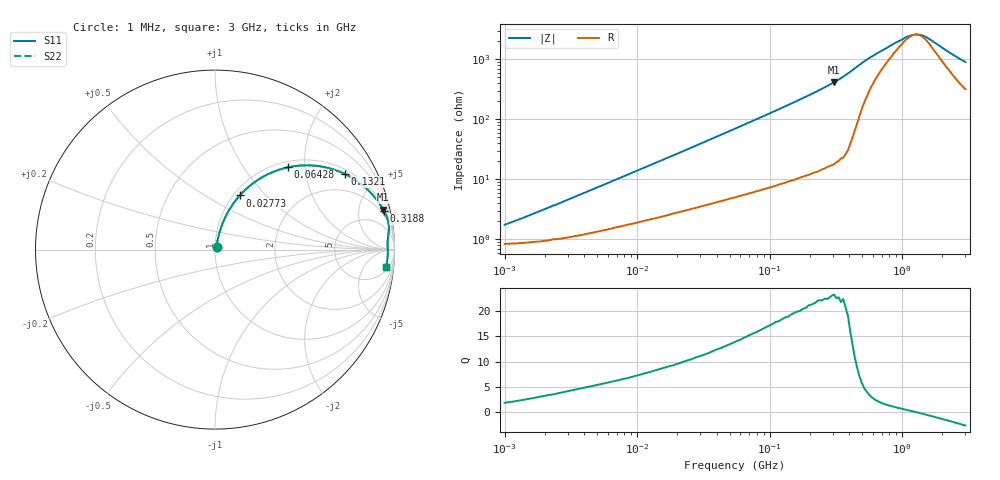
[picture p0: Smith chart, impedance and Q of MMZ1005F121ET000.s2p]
! S-parameter Generated by TDK Corporation
! Copyright(C) 2016 TDK Corporation.
! All Rights Reserved.
! TDK P/N: MMZ1005F121ET000 (Chip Beads)
! Property: |Z|=120¶ at 100MHz
! Size(LxWxT): 1x0.5x0.5mm, 0.039x0.02x0.02inches
! Model Type: s2p (Touchstone File Format Version 1.0)
! Frequency: DC=Yes Start=1MHz Stop=3000MHz 202points Log-sweep
! Note: This model was converted from impedance.
! Model Generated on May. 16, 2016
! Hash(MD5):
! Port Assignments:
!  1 ---@@@--- 2
! Applicable Conditions:
!  Temperature = 25 degC
!  DC Bias Current = 0 A
!  Small Signal Operation
! Terms and conditions regarding TDK Simulation Models
! (1)This simulation model is being provided solely for informational purposes. Please refer to the specifications of the products in terms of detailed characteristics of such products.
! (2)In no event shall TDK Corporation of any of its subsidiaries be liable for any loss or damage arising, directly or indirectly,
!  From any information contained in this simulation model, including, but not limited to loss or damages arising from any inaccuracies, omissions or errors in connection with such information.
! (3)Any and all copyrights on this simulation model are owned by TDK Corporation.
!  Duplication or redistribution of this simulation model without prior written permission from TDK Corporation is prohibited.
! (4)This simulation model is subject to any modification or change without any prior notice.
! (5)Neither TDK Corporation nor any of its subsidiaries shall make any warranty, express or implied,
!  Including but not limited to the correctness, implied warranties of merchantability and fitness for a particular purpose with respect to this simulation models.
! (6)The use of this simulation model shall be deemed to have consented to the terms and conditions hereof.
# MHz S MA R 50
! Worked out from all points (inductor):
!   201 points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, 1 MHz to 3 GHz, reference 50 ohm
!   read as one part in series: L = 240 nH near 1.823 MHz
!   highest Q = 22.7 at 306.3 MHz (marker M1), where L = 216 nH
!   self-resonance near 1.266 GHz
!   S11 on the Smith chart (normalised r, x): 1 MHz: 1.02, +0.03; 27.73 MHz: 1.07, +0.72; 64.28 MHz: 1.11, +1.63; 132.1 MHz: 1.18, +3.32; 318.8 MHz: 1.39, +8.72; 3 GHz: 7, -17
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1  0.01732 60.5  0.9916 -0.9  0.9916 -0.9  0.01732 60.5
3.900413  0.05746 74.9  0.9866 -3.2  0.9866 -3.2  0.05746 74.9
8.345207  0.1146 75.0  0.9766 -6.5  0.9766 -6.5  0.1146 75.0
14.61624  0.1903 72.4  0.9597 -10.9  0.9597 -10.9  0.1903 72.4
27.73354  0.3319 65.4  0.9132 -19.3  0.9132 -19.3  0.3319 65.4
39.76269  0.442 59.2  0.862 -26.1  0.862 -26.1  0.442 59.2
54.77226  0.554 52.3  0.7936 -33.5  0.7936 -33.5  0.554 52.3
64.28402  0.6118 48.5  0.7506 -37.6  0.7506 -37.6  0.6118 48.5
92.16659  0.7359 39.3  0.6346 -47.3  0.6346 -47.3  0.7359 39.3
132.1429  0.8372 30.2  0.5042 -56.7  0.5042 -56.7  0.8372 30.2
213.6344  0.9255 19.7  0.338 -67.6  0.338 -67.6  0.9255 19.7
306.2963  0.9628 13.4  0.2319 -74.1  0.2319 -74.1  0.9628 13.4
318.8066  0.9655 12.8  0.2212 -74.7  0.2212 -74.7  0.9655 12.8
389.4533  0.977 9.7  0.1681 -77.3  0.1681 -77.3  0.977 9.7
515.4121  0.9732 5.9  0.1056 -72.3  0.1056 -72.3  0.9732 5.9
800.5644  0.963 2.7  0.0586 -49.5  0.0586 -49.5  0.963 2.7
1102.76  0.9626 0.8  0.03997 -20.1  0.03997 -20.1  0.9626 0.8
1243.477  0.9627 0.1  0.03734 -2.6  0.03734 -2.6  0.9627 0.1
1402.151  0.9634 -0.6  0.03805 15.3  0.03805 15.3  0.9634 -0.6
1581.072  0.9633 -1.3  0.04319 31.2  0.04319 31.2  0.9633 -1.3
2359.433  0.9609 -3.9  0.07804 58.0  0.07804 58.0  0.9609 -3.9
3000  0.9576 -5.7  0.1062 63.7  0.1062 63.7  0.9576 -5.7
